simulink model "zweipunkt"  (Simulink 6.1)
settings: Solver=ode1  StartTime=0.0  StopTime=120  FixedStep=1e-3  RelTol=1e-3
libraries: simulink x1

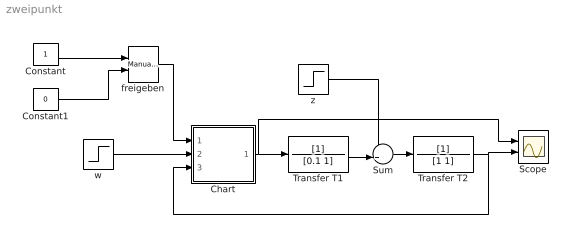
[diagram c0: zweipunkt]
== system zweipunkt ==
  Chart : Stateflow chart
  Constant : Constant
  Constant1 : Constant  Value=0
  Scope : Scope  NumInputPorts=2
  Sum : Sum  Inputs=-+|
  Transfer T1 : TransferFcn  Denominator=[0.1 1]
  Transfer T2 : TransferFcn  Denominator=[1 1]
  freigeben : simulink/Signal Routing/Manual Switch  sw=1  action=0
  w : Step  After=5  SampleTime=0
  z : Step  Time=60  After=2  SampleTime=0
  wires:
  Transfer T1/1 -> Sum/2
  Sum/1 -> Transfer T2/1
  Transfer T2/1 -> Chart/3(y), Scope/2
  z/1 -> Sum/1
  Chart/1(u) -> Transfer T1/1, Scope/1
  Constant1/1 -> freigeben/2
  Constant/1 -> freigeben/1
  freigeben/1 -> Chart/1(freigeben)
  w/1 -> Chart/2(w)

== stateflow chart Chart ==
  state blockiert/
    en: u=0;
  state Freigabe/
    during: on every(10,zaehlerevent): ml.zaehler++;
    state u0/
      en: u=0;
    state u10/
      en: u=10;
    (default) -> u0
    u0 -> u10 : [y<0.9*w]/zaehlerevent;
    u10 -> u0 : [y>1.1*w]
  blockiert -> Freigabe : [freigeben]
  Freigabe -> blockiert : [~freigeben]
  (default) -> blockiert : /ml.zaehler=0;
